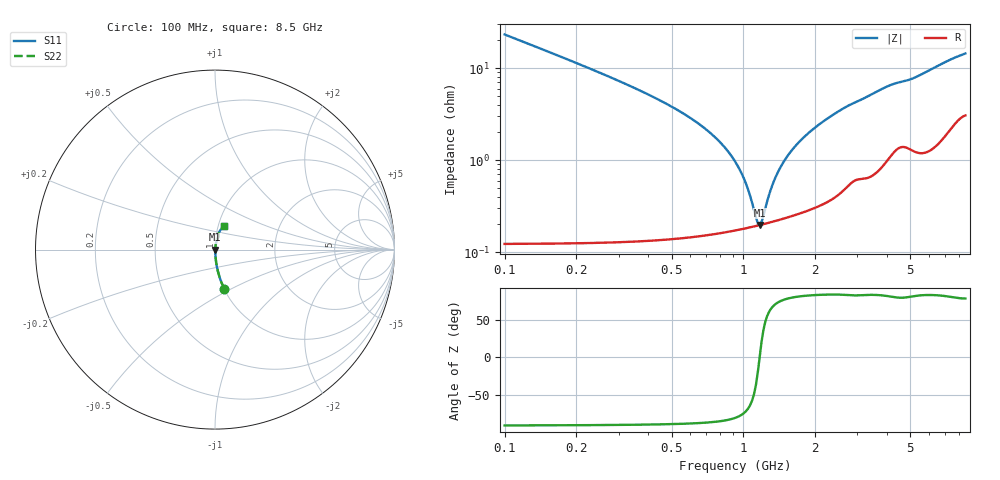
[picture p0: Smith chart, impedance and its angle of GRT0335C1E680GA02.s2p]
!Murata Part Number: GRT0335C1E680GA02
!These Parameters are Measured in Series Mode Connection
!Data Generated on Jun 19, 2026
!  o--ll--o
!Port1  Port2
!  o------o
!Operation Temp=25[degC], DC Bias Voltage=0[V]
!Freq. Start=100[MHz] Stop=9[GHz] 401[Steps]
# Hz S RI R 50
!Freq.(Hz) S11(Real) S11(Imag) S21(Real) S21(Imag) S12(Real) S12(Imag) S22(Real) S22(Imag)
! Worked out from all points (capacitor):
!   401 points, 100 MHz to 8.5 GHz, reference 50 ohm
!   read as one part in series: C = 68 pF near 142 MHz
!   lowest |Z| = 197 mohm at 1.171 GHz (marker M1)
!   series resonance near 1.169 GHz, so ESL is about 270 pH
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1e8  0.0523 -0.2199  0.9477 0.2199  0.9477 0.2199  0.0523 -0.2199
2.05e8  0.0133 -0.109  0.9867 0.109  0.9867 0.109  0.0133 -0.109
3.1e8  0.00616 -0.0696  0.9938 0.0696  0.9938 0.0696  0.00616 -0.0696
4.36e8  0.00346 -0.0459  0.9965 0.0459  0.9965 0.0459  0.00346 -0.0459
7.51e8  0.00189 -0.0182  0.9981 0.0182  0.9981 0.0182  0.00189 -0.0182
8.98e8  0.0018 -0.0106  0.9982 0.0106  0.9982 0.0106  0.0018 -0.0106
1.003e9  0.00183 -0.0061  0.9982 0.0061  0.9982 0.0061  0.00183 -0.0061
1.129e9  0.00192 -0.00137  0.9981 0.00137  0.9981 0.00137  0.00192 -0.00137
1.171e9  0.00197 7.68e-05  0.998 -7.68e-05  0.998 -7.68e-05  0.00197 7.68e-05
1.213e9  0.00201 0.00147  0.998 -0.00147  0.998 -0.00147  0.00201 0.00147
1.297e9  0.00212 0.00413  0.9979 -0.00413  0.9979 -0.00413  0.00212 0.00413
1.36e9  0.00221 0.00603  0.9978 -0.00603  0.9978 -0.00603  0.00221 0.00603
1.507e9  0.00245 0.0102  0.9975 -0.0102  0.9975 -0.0102  0.00245 0.0102
1.738e9  0.00291 0.0161  0.9971 -0.0161  0.9971 -0.0161  0.00291 0.0161
2.032e9  0.00362 0.0231  0.9964 -0.0231  0.9964 -0.0231  0.00362 0.0231
2.452e9  0.00507 0.0323  0.9949 -0.0323  0.9949 -0.0323  0.00507 0.0323
2.914e9  0.00762 0.0411  0.9924 -0.0411  0.9924 -0.0411  0.00762 0.0411
3.754e9  0.0113 0.0568  0.9887 -0.0568  0.9887 -0.0568  0.0113 0.0568
4.3e9  0.0166 0.065  0.9834 -0.065  0.9834 -0.065  0.0166 0.065
5.707e9  0.0192 0.085  0.9808 -0.085  0.9808 -0.085  0.0192 0.085
7.114e9  0.0317 0.1115  0.9683 -0.1115  0.9683 -0.1115  0.0317 0.1115
8.5e9  0.0476 0.1304  0.9524 -0.1304  0.9524 -0.1304  0.0476 0.1304
